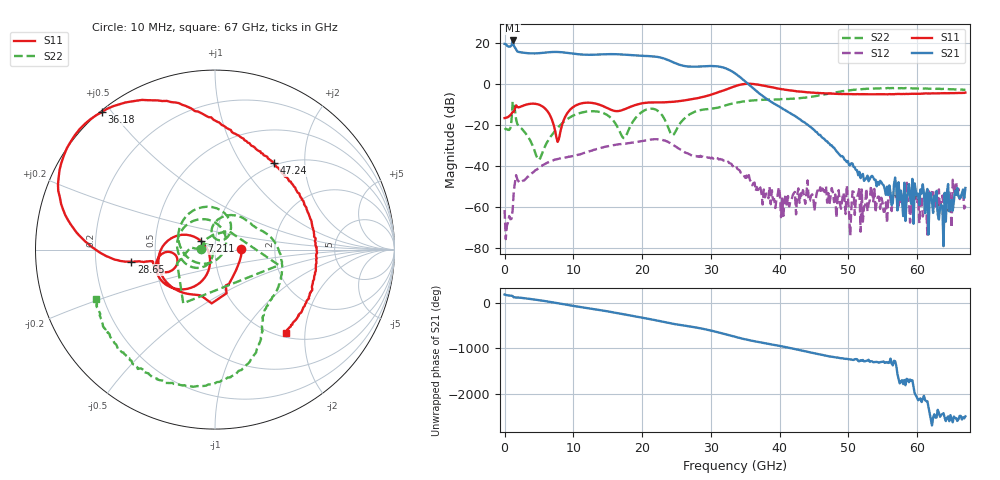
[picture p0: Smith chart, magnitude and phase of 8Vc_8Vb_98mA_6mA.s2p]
! MARKI MICROWAVE INC.
! Date:  05/05/2020
! Model Number:  APM-7099CH
! Description:  2-port Small Signal S-parameter data for APM-7099CH
! Frequency Range:  10 MHz to 67 GHz
! Port Configuration:  PORT 1: Input
!  PORT 2: Output
! Bias Condition: Vc = +8V, Vb = +8V
! APM-7099CH s2p files are only valid for small signal conditions (below -5 dBm input power)
!S2P File: Measurements: Mag<S11> Ang<S11>, Mag<S21> Ang<S21>, Mag<S12> Ang<S12>, Mag<S22> Ang<S22>!row 1
# Hz S  dB  R 50
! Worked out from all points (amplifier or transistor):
!   401 points, 10 MHz to 67 GHz, reference 50 ohm
!   highest |S21| = 21.2 dB at 1.182 GHz (marker M1)
!   |S21| within 3 dB of that: start of sweep to 646.5 MHz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
!   unconditionally stable (mu >= 1): start of sweep to 34.75 GHz; 36.13 GHz to end of sweep
!   at 11.06 GHz: K = 4.28, MAG = 15.0 dB, |S12| = -34.3 dB
!   at 33.51 GHz: K = 5.75, MAG = 12.2 dB, |S12| = -40.3 dB
!   at 67 GHz: K = 49011.07, MAG = -45.6 dB, |S12| = -59.4 dB
!   S11 on the Smith chart (normalised r, x): 10 MHz: 1.34, +0.01; 7.211 GHz: 0.85, +0.08; 28.65 GHz: 0.36, -0.06; 36.18 GHz: 0.00, +0.47; 47.24 GHz: 0.96, +1.41; 67 GHz: 1.07, -1.60
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1e7  -16.65 1.4  19.50 178.5  -61.54 150.2  -22.38 178.9
1.182325e9  -13.68 -68.1  21.18 143.8  -61.45 77.9  -8.72 -13.7
2.0197e9  -11.45 -108.1  15.60 112.1  -47.44 -116.9  -20.24 174.4
5.03425e9  -10.17 -176.1  14.97 54.9  -40.94 -178.7  -36.95 -158.3
7.211425e9  -20.89 148.5  15.58 1.8  -37.05 127.2  -23.45 -111.3
9.221125e9  -13.83 -114.4  15.08 -51.2  -35.64 84.5  -16.96 -134.0
1.123082e10  -9.46 -144.8  14.32 -98.9  -34.01 49.4  -13.97 -169.6
1.47478e10  -11.50 -177.3  14.46 176.4  -30.60 -22.4  -14.85 110.4
1.759488e10  -12.16 -155.5  14.22 98.9  -29.14 -87.6  -25.75 -67.6
2.027448e10  -9.32 -161.0  13.63 25.7  -27.75 -150.7  -13.05 156.1
2.245165e10  -9.06 -168.8  13.00 -40.5  -27.04 145.4  -13.54 75.1
2.362398e10  -8.94 -169.6  11.85 -77.7  -28.03 107.6  -19.81 45.1
2.513125e10  -8.51 -170.0  9.69 -118.7  -31.13 66.9  -21.47 100.0
2.864822e10  -6.54 -171.6  8.53 153.9  -35.61 12.3  -12.69 51.3
3.08254e10  -4.34 -176.6  8.59 79.7  -36.17 -30.1  -11.75 28.2
3.21652e10  -2.81 176.5  7.57 26.5  -37.83 -59.2  -10.45 17.2
3.3505e10  -1.15 165.2  5.16 -27.7  -40.31 -98.8  -9.26 4.9
3.61846e10  -0.07 129.4  -2.31 -120.1  -48.37 -160.9  -8.02 -20.4
4.472582e10  -4.25 69.6  -21.68 -17.7  -53.82 -17.8  -6.24 -57.3
4.723795e10  -4.68 56.0  -29.20 -97.9  -58.68 -108.0  -4.72 -65.1
5.594665e10  -4.97 6.3  -49.51 126.4  -51.27 -149.9  -2.09 -111.0
6.7e10  -4.26 -49.7  -50.77 31.5  -59.38 -163.1  -2.90 -157.3
